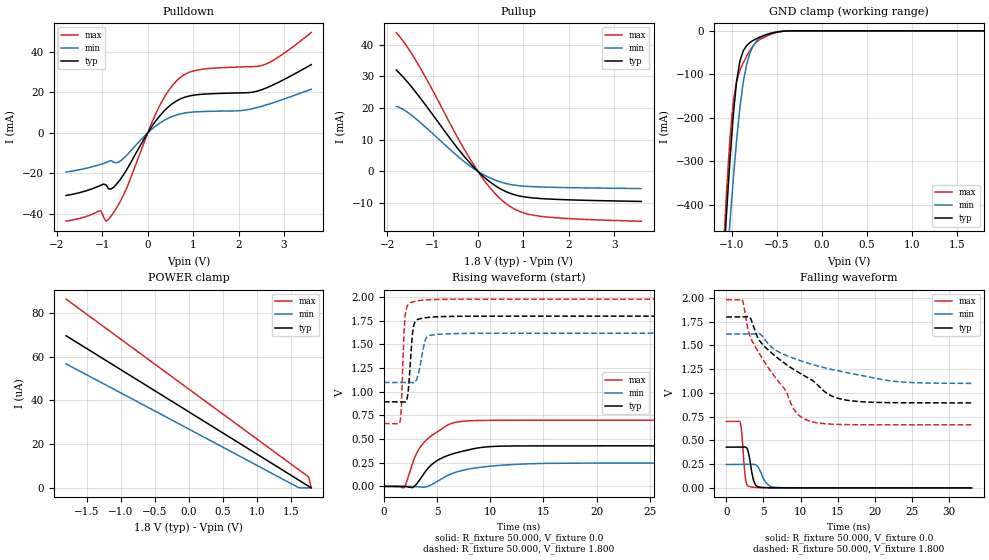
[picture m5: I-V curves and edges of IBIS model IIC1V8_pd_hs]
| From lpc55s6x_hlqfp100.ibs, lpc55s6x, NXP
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|   Model IIC1V8_pd_hs
[Model] IIC1V8_pd_hs
Model_type I/O
Polarity   Non-Inverting
Enable   Active-Low
Vinl =  0.540V
Vinh =  1.260V
Vmeas =  0.900V
Cref =  0.0F
Rref =  100.000
Vref =  0.0V
C_comp   2.515pF   2.512pF   2.535pF
C_comp_pullup   0.454pF   0.388pF   0.547pF
C_comp_pulldown   1.736pF   1.670pF   1.792pF
[Model Spec]
Vinh   1.260V   1.134V   1.386V
Vinl   0.540V   0.486V   0.594V
Vmeas   0.900V   0.810V   0.990V
Vref   0.0V   0.0V   0.0V
Cref   0.0F   0.0F   0.0F
Rref   1000.000   1000.000   1000.000
[Temperature Range]   25.000   0.125k   -40.000
[Voltage Range]   1.800V   1.620V   1.980V
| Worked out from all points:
|   slope of the pulldown table from 0 to 0.27 V, typ, clamps not added: 31.5 ohm
|   slope of the pullup table from 0 to 0.27 V, typ, clamps not added: 79.6 ohm
|   GND clamp passes 1 mA (typ) near -0.44 V on its own axis
|   rising waveform, R_fixture 50.000, V_fixture 0.0: 20-80 % time 2.97ns typ, 3.78ns min, 2.39ns max; typ from 0 V to 0.429 V
|   rising waveform, R_fixture 50.000, V_fixture 1.800: 20-80 % time 348ps typ, 536ps min, 254ps max; typ from 0.894 V to 1.8 V
|   falling waveform, R_fixture 50.000, V_fixture 0.0: 20-80 % time 598ps typ, 964ps min, 409ps max; typ from 0.429 V to 0 V
|   falling waveform, R_fixture 50.000, V_fixture 1.800: 20-80 % time 8.37ns typ, 11.2ns min, 5.71ns max; typ from 1.8 V to 0.894 V
[Pulldown]
|Voltage   I(typ)   I(min)   I(max)
-1.8V     -30.97mA   -19.41mA   -43.61mA
-1.03V    -25.91mA   -15.56mA   -38.59mA
-920mV    -25.75mA   -14.67mA   -43.75mA
-865mV    -27.69mA   -14.16mA   -42.79mA
-700mV    -25.69mA   -14.87mA   -37.58mA
-480mV    -18.8mA    -11.48mA   -28.03mA
235mV     7.619mA    4.356mA    12.23mA
455mV     12.83mA    7.267mA    20.76mA
730mV     16.88mA    9.427mA    27.6mA
1.17V     19mA       10.49mA    31.33mA
2.545V    21.61mA    13.36mA    33.53mA
3.6V      33.71mA    21.52mA    49.57mA
[Pullup]
|Voltage   I(typ)   I(min)   I(max)
-1.8V     32.05mA    20.54mA    43.88mA
-1.57V    28.56mA    18.87mA    39.61mA
-1.295V   23.65mA    15.76mA    33.3mA
-1.02V    18.4mA     12.24mA    26.22mA
-470mV    7.714mA    5.076mA    11.29mA
-30mV     432.2uA    271.3uA    660.2uA
300mV     -3.713mA   -2.28mA    -5.781mA
630mV     -6.475mA   -3.874mA   -10.31mA
960mV     -7.909mA   -4.606mA   -12.9mA
1.4V      -8.61mA    -4.943mA   -14.23mA
2.17V     -9.075mA   -5.188mA   -15.07mA
3.6V      -9.515mA   -5.442mA   -15.79mA
[GND_clamp]
|Voltage   I(typ)   I(min)   I(max)
-1.8V     -3.488A    -3.23A     -3.872A
-1.097V   -545.5mA   -658.5mA   -507mA
-1.06V    -414.6mA   -546.1mA   -365mA
-1.023V   -294.9mA   -439.1mA   -245.9mA
-986mV    -192.4mA   -339.6mA   -162mA
-949mV    -115.6mA   -250.3mA   -115.1mA
-912mV    -69.19mA   -175.2mA   -90.62mA
-838mV    -34.02mA   -77.16mA   -58.5mA
-764mV    -21.82mA   -34.11mA   -33.6mA
-653mV    -11.43mA   -11.65mA   -15.83mA
-431mV    -835.3uA   -879.6uA   -1.141mA
1.8V      0A         0A         0A
[POWER_clamp]
|Voltage   I(typ)   I(min)   I(max)
-1.8V     69.55uA    56.68uA    86.29uA
1.615V    3.579uA    80.87nA    8.337uA
1.763V    715.6nA    0A         4.957uA
1.8V      0A         0A         0A
[Ramp]
| variable   typ   min   max
dV/dt_r   0.257/2.973n   0.148/3.773n   0.419/2.390n
dV/dt_f   0.543/8.367n   0.311/11.166n   0.789/5.707n
R_load = 50.000
[Rising Waveform]
R_fixture= 50.000
V_fixture= 0.0
V_fixture_min= 0.0
V_fixture_max= 0.0
|time   V(typ)   V(min)   V(max)
0s        6.59nV     69.96nV    4.613nV
1.899ns   194.8uV    -157.7nV   -12.49mV
2.768ns   -9.17mV    -28.49uV   270mV
3.587ns   107.2mV    -8.164mV   441mV
4.859ns   262.4mV    41.97mV    565.1mV
6.007ns   326.6mV    116.8mV    649.1mV
6.837ns   355.9mV    152.5mV    679.1mV
9.477ns   415.6mV    207.4mV    697.4mV
13.66ns   428mV      238.9mV    698.9mV
33ns      428.6mV    246.2mV    699.1mV
[Rising Waveform]
R_fixture= 50.000
V_fixture= 1.800
V_fixture_min= 1.620
V_fixture_max= 1.980
|time   V(typ)   V(min)   V(max)
0s        893.8mV    1.098V     663mV
1.518ns   893.8mV    1.098V     688.5mV
1.645ns   893.9mV    1.098V     853.4mV
1.967ns   891.1mV    1.098V     1.774V
2.279ns   1.003V     1.099V     1.922V
2.63ns    1.552V     1.096V     1.948V
2.983ns   1.747V     1.112V     1.958V
3.884ns   1.782V     1.546V     1.971V
4.451ns   1.789V     1.6V       1.974V
33ns      1.799V     1.619V     1.979V
[Falling Waveform]
R_fixture= 50.000
V_fixture= 0.0
V_fixture_min= 0.0
V_fixture_max= 0.0
|time   V(typ)   V(min)   V(max)
0s        428.7mV    246.3mV    699.2mV
1.87ns    428.7mV    246.3mV    689.5mV
2.082ns   428.6mV    246.3mV    574.3mV
2.555ns   430.4mV    246.3mV    109.6mV
3.067ns   336.8mV    246.3mV    13.81mV
3.681ns   77.49mV    247.6mV    5.765mV
4.445ns   7.612mV    197.2mV    2.189mV
5.381ns   2.553mV    51.85mV    818.6uV
6.461ns   979.1uV    5.202mV    303.6uV
33ns      945.6nV    1.919uV    548.8nV
[Falling Waveform]
R_fixture= 50.000
V_fixture= 1.800
V_fixture_min= 1.620
V_fixture_max= 1.980
|time   V(typ)   V(min)   V(max)
0s        1.799V     1.619V     1.979V
2.132ns   1.799V     1.619V     1.983V
2.93ns    1.805V     1.619V     1.661V
3.529ns   1.729V     1.619V     1.538V
5.09ns    1.492V     1.571V     1.332V
7.968ns   1.304V     1.398V     1.026V
9.228ns   1.239V     1.359V     812.2mV
10.48ns   1.181V     1.325V     726.7mV
16.17ns   923.1mV    1.214V     665.9mV
33ns      894.3mV    1.1V       663.2mV
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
